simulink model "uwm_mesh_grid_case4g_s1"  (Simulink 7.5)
settings: Solver=ode45  StartTime=0.0  StopTime=8.0  RelTol=1e-4
undefined symbols (not defined in the file or in its folder): D1, Delta, dfilt, DiscIntNeverNeededParam
libraries: powerlib x90, powerlib_extras x24, dsparch4 x6
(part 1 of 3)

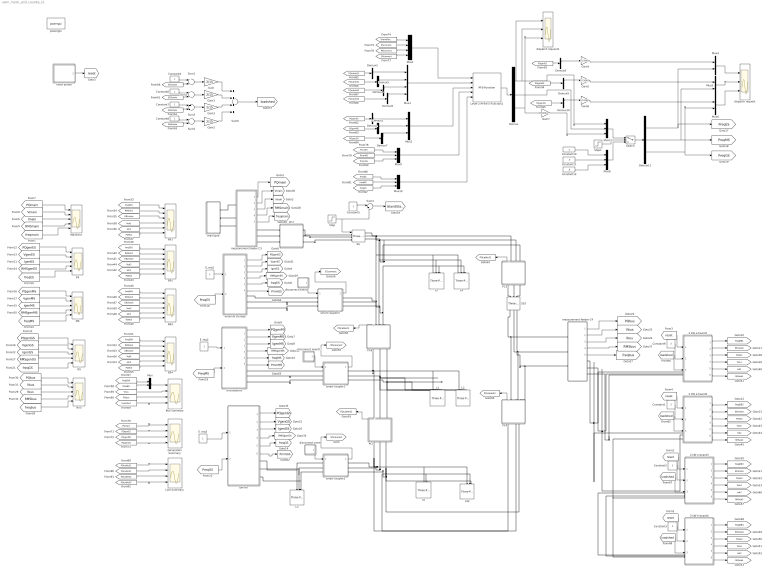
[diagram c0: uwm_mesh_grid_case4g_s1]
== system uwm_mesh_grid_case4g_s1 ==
  2 kW e-board1 : Subsystem
  2 kW e-board2 : Subsystem
  2 kW e-board3 : Subsystem
  2 kW e-board4 : Subsystem
  BUS : Scope  NumInputPorts=5
  Bus Summary : Scope  NumInputPorts=4
  Constant{1..3,9} (4 alike) : Constant  Value=2  OutDataType=fixdt(1, 16)  OutScaling=2^0
  Constant10 : Constant  Value=-.1  OutDataType=fixdt(1, 16)  OutScaling=2^0
  Constant11 : Constant  Value=.5  OutDataType=fixdt(1, 16)  OutScaling=2^0
  Constant12 : Constant  Value=.8  OutDataType=fixdt(1, 16)  OutScaling=2^0
  Constant{4..8} (5 alike) : Constant  OutDataType=fixdt(1, 16)  OutScaling=2^0
  Demux : Demux  Outputs=3
  Demux{1..10} (10 alike) : Demux  Outputs=2
  Demux11 : Demux  Outputs=3
  EB{1..4} (4 alike) : Scope  NumInputPorts=6
  ES : Scope  NumInputPorts=5
  E_req1 : Constant  OutDataType=fixdt(1, 16)  OutScaling=2^0
  E_req2 : Constant  OutDataType=fixdt(1, 16)  OutScaling=2^0
  E_req3 : Constant  OutDataType=fixdt(1, 16)  OutScaling=2^0
  GS : Scope  NumInputPorts=5
  Gain{,1..3} (4 alike) : Gain  Gain=2/15  ParameterDataType=fixdt(1, 16)  ParameterScaling=2^0  OutDataType=fixdt(1, 16)  OutScaling=2^0
  Gain4 : Gain  Gain=1/15000  ParameterDataType=fixdt(1, 16)  ParameterScaling=2^0  OutDataType=fixdt(1, 16)  OutScaling=2^0
  Gain5 : Gain  Gain=1/15000  ParameterDataType=fixdt(1, 16)  ParameterScaling=2^0  OutDataType=fixdt(1, 16)  OutScaling=2^0
  Gain6 : Gain  Gain=1/12500  ParameterDataType=fixdt(1, 16)  ParameterScaling=2^0  OutDataType=fixdt(1, 16)  OutScaling=2^0
  Gain7 : Gain  Gain=15000/12500  ParameterDataType=fixdt(1, 16)  ParameterScaling=2^0  OutDataType=fixdt(1, 16)  OutScaling=2^0
  Generation Summary : Scope  NumInputPorts=4
  L{1..4,42} (5 alike) : powerlib/Elements/Three-Phase Series RLC Load  DialogController=POWERSYS.PowerSysDialog  PhysicalDomain=powersysdomain  SubClassName=unknown  LeftPortType=p1  RightPortType=p1  LConnTagsString=A|B|C  Configuration=Y (grounded)  NominalVoltage=208  NominalFrequency=60  ActivePower=4000  InductivePower=0  CapacitivePower=0  Measurements=None
  L5 : powerlib/Elements/Three-Phase Series RLC Load  DialogController=POWERSYS.PowerSysDialog  PhysicalDomain=powersysdomain  SubClassName=unknown  LeftPortType=p1  RightPortType=p1  LConnTagsString=A|B|C  Configuration=Y (grounded)  NominalVoltage=208  NominalFrequency=60  ActivePower=2000  InductivePower=0  CapacitivePower=0  Measurements=None
  L6 : powerlib/Elements/Three-Phase Series RLC Load  DialogController=POWERSYS.PowerSysDialog  PhysicalDomain=powersysdomain  SubClassName=unknown  LeftPortType=p1  RightPortType=p1  LConnTagsString=A|B|C  Configuration=Y (grounded)  NominalVoltage=208  NominalFrequency=60  ActivePower=2000  InductivePower=0  CapacitivePower=0  Measurements=None
  Level-2 M-file S-Function1 : M-S-Function  FunctionName=dispatcher3
  Line Summary : Scope  NumInputPorts=4
  MS : Scope  NumInputPorts=5
  MainGrid : Scope  NumInputPorts=5
  Mux{,4..6} (4 alike) : Mux  Inputs=2
  Mux1 : Mux
  Mux{2,7..10} (5 alike) : Mux  Inputs=3
  Mux3 : Mux
  PC2 : Subsystem  mask{R=.002810, L=.000679, C=2894.3}
  PC3 : Subsystem  mask{R=0.027352, L=.006600, C=288.6}
  PC4 : Subsystem  mask{R=.01688, L=.004070, C=336.7}
  PC5 : Subsystem  mask{R=.002600, L=.000640, C=2020.1}
  PC6 : Subsystem  mask{R=.013700, L=.003300, C=577.2}
  SS : powerlib/Elements/Three-Phase Breaker  DialogController=POWERSYS.PowerSysDialog  SystemSampleTime=-1  InitialState=closed  SwitchA=on  SwitchB=on  SwitchC=on  SwitchTimes=[1.]  External=on  BreakerResistance=.001  SnubberResistance=1e6  SnubberCapacitance=inf  Measurements=None
  SS3 : powerlib/Elements/Three-Phase Breaker  DialogController=POWERSYS.PowerSysDialog  SystemSampleTime=-1  InitialState=closed  SwitchA=on  SwitchB=on  SwitchC=on  SwitchTimes=[50]  External=off  BreakerResistance=.00001  SnubberResistance=1e10  SnubberCapacitance=inf  Measurements=None
  Step : Step  Before=1  After=0  SampleTime=0
  Step1 : Step  Time=100  SampleTime=0
  Sum{1..3,5} (4 alike) : Sum  Inputs=+-  OutDataType=fixdt(1, 16)  OutScaling=2^0
  Sum4 : Sum  Inputs=|+-  OutDataType=fixdt(1, 16)  OutScaling=2^0
  Sum6 : Sum  Inputs=++++  OutDataType=fixdt(1, 16)  OutScaling=2^0
  Switch : Switch  Threshold=1/2  OutDataType=fixdt(1, 16)  OutScaling=2^0
  disconnect event : Subsystem  mask{tstart=50, tstop=60}
      mask prompts: tstart "disconnect time"; tstop "connect time"
  disconnect event1 : Subsystem  mask{tstart=3.0, tstop=3.5}
      mask prompts: tstart "disconnect time"; tstop "connect time"
  disconnect event2 : Subsystem  mask{tstart=50, tstop=60}
      mask prompts: tstart "disconnect time"; tstop "connect time"
  dispatch request : Scope  NumInputPorts=3
  dispatch request1 : Scope  NumInputPorts=3
  external storage : Subsystem  AncestorBlock=|
      | UWM_blocks/inverter-based
      | DG (simplified)
      | 208V - 15kVA
  genset : Subsystem
  main grid : Subsystem
  measurement feeder C3 : Subsystem
  measurement feeder C4 : Subsystem
  microsource : Subsystem  AncestorBlock=|
      | UWM_blocks/inverter-based
      | DG (simplified)
      | 208V - 15kVA
  powergui : powerlib/powergui  Priority=1  SystemSampleTime=-1  SimulationMode=Discrete  SampleTime=20e-6  frequency=60  SPID=off  DisableSnubberDevices=off  DisableRonSwitches=off  DisableVfSwitches=off  SwTol=0  Interpol=off  frequencyindice=60  echomessages=off  HookPort=off  DisplayEquations=off  FunctionMessages=off  EnableUseOfTLC=off  x0status=steady  RestoreLinks=no  ResistiveCurrentMeasurement=off  Frange=[0:2:500]  Ylog=off  Xlog=on  ShowGrid=off  save=off  variable=ZData  ZoomFFT=on  StartTime=0.0  cycles=1  DisplayStyle=1  fundamental=60  FreqAxis=off  MaxFrequency=1000  frequencyindicesteady=1  RmsSteady=2  display=off  Ts=0  methode=off
  reset pulses : Subsystem  mask{tpulse=[50 100]}
  smart coupler1 : Subsystem
  smart coupler2 : Subsystem
  smart coupler3 : Subsystem
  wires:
  [PreqMS] -> microsource/2(P_req)
  E_req2/1 -> microsource/1(E_req)
  E_req1/1 -> external storage/1(E_req)
  E_req3/1 -> genset/1(Ereq)
  [PreqGS] -> genset/2(Preq)
  reset pulses/1(Out1) -> [reset]
  2 kW e-board1/1(w) -> [freqEB1]
  2 kW e-board1/2(state) -> [EB1state]
  measurement feeder C3/3(I) -> [Imain]
  measurement feeder C3/1(PQ) -> [PQmain]
  [PreqES] -> external storage/2(P_req)
  measurement feeder C3/2(V) -> [Vmain]
  [PQmain] -> MainGrid/1
  [Vmain] -> MainGrid/2
  [Imain] -> MainGrid/3
  [RMSmain] -> MainGrid/4
  external storage/5(freq) -> [freqES]
  external storage/3(I) -> [IgenES]
  external storage/2(V) -> [VgenES]
  external storage/1(PQ) -> [PQgenES]
  microsource/1(PQ) -> [PQgenMS]
  microsource/2(V) -> [VgenMS]
  microsource/3(I) -> [IgenMS]
  microsource/5(freq) -> [freqMS]
  genset/1(PQ) -> [PQgenGS]
  genset/2(V) -> [VgenGS]
  genset/3(I) -> [IgenGS]
  genset/5(freq) -> [freqGS]
  measurement feeder C4/1(PQ) -> [PQbus]
  measurement feeder C4/2(V) -> [Vbus]
  measurement feeder C4/3(I) -> [Ibus]
  measurement feeder C4/5(freq) -> [freqbus]
  measurement feeder C3/4(RMS) -> [RMSmain]
  external storage/4(RMS) -> [RMSgenES]
  microsource/4(RMS) -> [RMSgenMS]
  genset/4(RMS) -> [RMSgenGS]
  measurement feeder C3/5(freq) -> [freqmain]
  [freqmain] -> MainGrid/5
  [PQgenES] -> ES/1
  [VgenES] -> ES/2
  [IgenES] -> ES/3
  [RMSgenES] -> ES/4
  [freqES] -> ES/5
  [PQgenMS] -> MS/1
  [VgenMS] -> MS/2
  [IgenMS] -> MS/3
  [RMSgenMS] -> MS/4
  [freqMS] -> MS/5
  [PQgenGS] -> GS/1
  [VgenGS] -> GS/2
  [IgenGS] -> GS/3
  [RMSgenGS] -> GS/4
  [freqGS] -> GS/5
  measurement feeder C4/4(RMS) -> [RMSbus]
  [PQbus] -> BUS/1
  [Vbus] -> BUS/2
  [Ibus] -> BUS/3
  [RMSbus] -> BUS/4
  [freqbus] -> BUS/5
  [freqEB1] -> EB1/1
  [RMSeb1] -> EB1/2
  [EB1state] -> EB1/3
  2 kW e-board1/3(PQ) -> [PQeb1]
  2 kW e-board1/4(V) -> [Veb1]
  2 kW e-board1/5(I) -> [Ieb1]
  2 kW e-board1/6(RMS) -> [RMSeb1]
  [PQeb1] -> EB1/6
  [Ieb1] -> EB1/5
  [Veb1] -> EB1/4
  [reset] -> 2 kW e-board2/1(reset)
  2 kW e-board2/1(w) -> [freqEB2]
  2 kW e-board2/2(state) -> [EB2state]
  Constant1/1 -> 2 kW e-board2/2(priority)
  2 kW e-board2/3(PQ) -> [PQeb2]
  2 kW e-board2/4(V) -> [Veb2]
  2 kW e-board2/5(I) -> [Ieb2]
  2 kW e-board2/6(RMS) -> [RMSeb2]
  2 kW e-board3/1(w) -> [freqEB3]
  2 kW e-board3/2(state) -> [EB3state]
  2 kW e-board3/3(PQ) -> [PQeb3]
  2 kW e-board3/4(V) -> [Veb3]
  2 kW e-board3/5(I) -> [Ieb3]
  2 kW e-board3/6(RMS) -> [RMSeb3]
  2 kW e-board4/1(w) -> [freqEB4]
  2 kW e-board4/2(state) -> [EB4state]
  2 kW e-board4/3(PQ) -> [PQeb4]
  2 kW e-board4/4(V) -> [Veb4]
  2 kW e-board4/5(I) -> [Ieb4]
  2 kW e-board4/6(RMS) -> [RMSeb4]
  [freqEB2] -> EB2/1
  [RMSeb2] -> EB2/2
  [EB2state] -> EB2/3
  [PQeb2] -> EB2/6
  [Ieb2] -> EB2/5
  [Veb2] -> EB2/4
  [freqEB3] -> EB3/1
  [RMSeb3] -> EB3/2
  [EB3state] -> EB3/3
  [PQeb3] -> EB3/6
  [Ieb3] -> EB3/5
  [Veb3] -> EB3/4
  [freqEB4] -> EB4/1
  [RMSeb4] -> EB4/2
  [EB4state] -> EB4/3
  [PQeb4] -> EB4/6
  [Ieb4] -> EB4/5
  [Veb4] -> EB4/4
  Step/1 -> SS/1, Sum4/2
  [freqEB4] -> Mux/1
  [freqES] -> Mux/2
  [PQbus] -> Bus Summary/3
  Mux/1 -> Bus Summary/1
  [Vbus] -> Bus Summary/2
  disconnect event/1(Out1) -> smart coupler2/1(event)
  smart coupler2/1(connected) -> [GSconnect]
  Constant5/1 -> Sum4/1
  Sum4/1 -> [IslandState]
  disconnect event1/1(Out1) -> smart coupler1/1(event)
  smart coupler1/1(connected) -> [MSconnect]
  disconnect event2/1(Out1) -> smart coupler3/1(event)
  smart coupler3/1(connected) -> [ESconnect]
  Constant4/1 -> Sum1/1
  [EB1state] -> Sum1/2
  Constant6/1 -> Sum2/1
  [EB2state] -> Sum2/2
  Constant7/1 -> Sum3/1
  [EB3state] -> Sum3/2
  Constant8/1 -> Sum5/1
  [EB4state] -> Sum5/2
  Sum1/1 -> Gain/1
  Sum2/1 -> Gain1/1
  Sum3/1 -> Gain3/1
  Sum5/1 -> Gain2/1
  Gain1/1 -> Sum6/2
  Gain3/1 -> Sum6/3
  Gain/1 -> Sum6/1
  Gain2/1 -> Sum6/4
  Sum6/1 -> [loadshed]
  [loadshed] -> 2 kW e-board2/3(shed_load)
  [reset] -> 2 kW e-board1/1(reset)
  Constant9/1 -> 2 kW e-board1/2(priority)
  [loadshed] -> 2 kW e-board1/3(shed_load)
  [reset] -> 2 kW e-board3/1(reset)
  Constant2/1 -> 2 kW e-board3/2(priority)
  [loadshed] -> 2 kW e-board3/3(shed_load)
  [reset] -> 2 kW e-board4/1(reset)
  Constant3/1 -> 2 kW e-board4/2(priority)
  [loadshed] -> 2 kW e-board4/3(shed_load)
  [loadshed] -> Bus Summary/4
  [PQgenES] -> Generation Summary/2
  [PQgenMS] -> Generation Summary/3
  [PQmain] -> Generation Summary/1
  [PQgenGS] -> Generation Summary/4
  [GSconnect] -> Mux1/4
  [MSconnect] -> Mux1/3
  [ESconnect] -> Mux1/2
  [IslandState] -> Mux1/1
  PC6/1(PQ) -> [PQcable21]
  PC5/1(PQ) -> [PQcable42]
  PC4/1(PQ) -> [PQcable43]
  PC3/1(PQ) -> [PQcable31]
  [PQcable31] -> Demux4/1
  [PQcable42] -> Demux5/1
  [PQcable21] -> Demux3/1
  [PQcable43] -> Demux6/1
  Demux3/1 -> Mux3/1
  Demux4/1 -> Mux3/2
  Demux5/1 -> Mux3/3
  Demux6/1 -> Mux3/4
  Mux1/1 -> Level-2 M-file S-Function1/1
  Mux3/1 -> Level-2 M-file S-Function1/2
  Level-2 M-file S-Function1/1 -> Demux/1
  [PQgenMS] -> Demux2/1
  [PQgenGS] -> Demux7/1
  [PQgenES] -> Demux1/1
  Mux2/1 -> Level-2 M-file S-Function1/3
  [PQcable21] -> Line Summary/1
  [PQcable31] -> Line Summary/2
  [PQcable42] -> Line Summary/3
  [PQcable43] -> Line Summary/4
  [PQgenMS] -> Demux9/1
  [PQgenGS] -> Demux10/1
  [PQgenES] -> Demux8/1
  Demux/1 -> dispatch request1/1, Mux7/1, dispatch request1/2
  Demux/2 -> Mux7/2
  Demux8/1 -> Gain4/1
  Gain4/1 -> Mux4/1
  Demux9/1 -> Gain5/1
  Gain5/1 -> Mux5/1
  Demux10/1 -> Gain6/1
  Gain6/1 -> Mux6/1
  Constant10/1 -> Mux8/1
  Constant11/1 -> Mux8/2
  Constant12/1 -> Mux8/3
  Mux8/1 -> Switch/3
  Mux7/1 -> Switch/1
  Switch/1 -> Demux11/1
  Step1/1 -> Switch/2
  genset/6(Pmm) -> [PmmGS]
  microsource/6(Pmm) -> [PmmMS]
  external storage/6(Pmm) -> [PmmES]
  [PmmES] -> Mux9/1
  [PmmMS] -> Mux9/2
  [PmmGS] -> Mux9/3
  Mux9/1 -> Level-2 M-file S-Function1/4
  Demux11/1 -> [PreqES], Mux4/2
  Demux11/2 -> [PreqMS], Mux5/2
  Demux11/3 -> [PreqGS], Mux6/2
  Mux4/1 -> dispatch request/1
  Mux5/1 -> dispatch request/2
  Mux6/1 -> dispatch request/3
  Demux/3 -> Gain7/1, dispatch request1/3
  Gain7/1 -> Mux7/3
  Demux1/1 -> Mux2/1
  Demux2/1 -> Mux2/2
  Demux7/1 -> Mux2/3
  [freqES] -> Mux10/1
  [freqMS] -> Mux10/2
  [freqGS] -> Mux10/3
  Mux10/1 -> Level-2 M-file S-Function1/5
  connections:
  measurement feeder C4/LConn1 -- PC4/RConn1 -- SS3/RConn1
  measurement feeder C4/LConn2 -- PC4/RConn2 -- SS3/RConn2
  measurement feeder C4/LConn3 -- PC4/RConn3 -- SS3/RConn3
  L42/LConn1 -- PC5/LConn1 -- PC4/LConn1 -- smart coupler2/RConn1 -- L6/LConn1
  L42/LConn3 -- PC4/LConn3 -- PC5/LConn3 -- smart coupler2/RConn3 -- L6/LConn3
  PC5/RConn1 -- L1/LConn1 -- L2/LConn1 -- PC6/LConn1 -- smart coupler1/RConn1
  L2/LConn2 -- L1/LConn2 -- PC5/RConn2 -- PC6/LConn2 -- smart coupler1/RConn2
  L2/LConn3 -- L1/LConn3 -- PC5/RConn3 -- PC6/LConn3 -- smart coupler1/RConn3
  main grid/RConn2 -- measurement feeder C3/LConn2
  main grid/RConn1 -- measurement feeder C3/LConn1
  measurement feeder C3/LConn3 -- main grid/RConn3
  measurement feeder C3/RConn1 -- PC2/LConn1
  measurement feeder C3/RConn2 -- PC2/LConn2
  measurement feeder C3/RConn3 -- PC2/LConn3
  PC2/RConn2 -- SS/LConn2
  PC2/RConn1 -- SS/LConn1
  SS/LConn3 -- PC2/RConn3
  SS3/LConn2 -- PC3/LConn2
  SS3/LConn3 -- PC3/LConn3
  SS3/LConn1 -- PC3/LConn1
  L5/LConn1 -- genset/RConn1 -- smart coupler2/LConn1
  L5/LConn2 -- genset/RConn2 -- smart coupler2/LConn2
  L5/LConn3 -- genset/RConn3 -- smart coupler2/LConn3
  2 kW e-board4/LConn2 -- measurement feeder C4/RConn2 -- 2 kW e-board1/LConn2 -- 2 kW e-board2/LConn2 -- 2 kW e-board3/LConn2
  2 kW e-board3/LConn3 -- measurement feeder C4/RConn3 -- 2 kW e-board1/LConn3 -- 2 kW e-board2/LConn3 -- 2 kW e-board4/LConn3
  2 kW e-board4/LConn1 -- measurement feeder C4/RConn1 -- 2 kW e-board1/LConn1 -- 2 kW e-board2/LConn1 -- 2 kW e-board3/LConn1
  PC6/RConn1 -- L3/LConn1 -- L4/LConn1 -- SS/RConn1 -- PC3/RConn1 -- smart coupler3/RConn1
  PC6/RConn2 -- L3/LConn2 -- L4/LConn2 -- SS/RConn2 -- PC3/RConn2 -- smart coupler3/RConn2
  PC6/RConn3 -- L3/LConn3 -- L4/LConn3 -- SS/RConn3 -- PC3/RConn3 -- smart coupler3/RConn3
  L42/LConn2 -- PC5/LConn2 -- smart coupler2/RConn2 -- PC4/LConn2 -- L6/LConn2
  microsource/RConn1 -- smart coupler1/LConn1
  smart coupler1/LConn2 -- microsource/RConn2
  smart coupler1/LConn3 -- microsource/RConn3
  smart coupler3/LConn1 -- external storage/RConn1
  smart coupler3/LConn2 -- external storage/RConn2
  smart coupler3/LConn3 -- external storage/RConn3

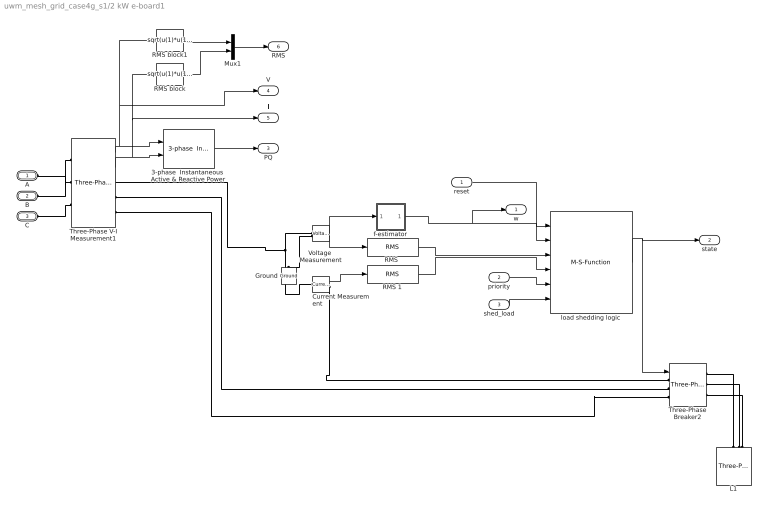
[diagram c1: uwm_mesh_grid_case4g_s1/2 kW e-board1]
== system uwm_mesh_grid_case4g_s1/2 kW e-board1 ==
  reset : Inport
  priority : Inport  Port=2
  shed_load : Inport  Port=3
  3-phase  Instantaneous  Active & Reactive Power : powerlib_extras/Measurements/3-phase  Instantaneous  Active & Reactive Power  DialogController=POWERSYS.PowerSysDialog  SystemSampleTime=-1
  Current Measurement : powerlib/Measurements/Current Measurement  DialogController=POWERSYS.PowerSysDialog  SystemSampleTime=-1  PhasorSimulation=off  OutputType=Complex  PSBequivalent=0
  Ground : powerlib/Elements/Ground  DialogController=POWERSYS.PowerSysDialog  PhysicalDomain=powersysdomain  SubClassName=unknown  LeftPortType=p1  RightPortType=p1  LConnTagsString=a
  L1 : powerlib/Elements/Three-Phase Series RLC Load  DialogController=POWERSYS.PowerSysDialog  PhysicalDomain=powersysdomain  SubClassName=unknown  LeftPortType=p1  RightPortType=p1  LConnTagsString=A|B|C  Configuration=Y (grounded)  NominalVoltage=208  NominalFrequency=60  ActivePower=2000  InductivePower=0  CapacitivePower=0  Measurements=None
  Mux1 : Mux  Inputs=2
  "RMS " : powerlib_extras/Measurements/RMS  DialogController=POWERSYS.PowerSysDialog  SystemSampleTime=-1  f1=60
  RMS 1 : powerlib_extras/Measurements/RMS  DialogController=POWERSYS.PowerSysDialog  SystemSampleTime=-1  f1=60
  RMS block : Fcn  Expr=sqrt(u(1)*u(1)+u(2)*u(2)+u(3)*u(3))/sqrt(3)
  RMS block1 : Fcn  Expr=sqrt(u(1)*u(1)+u(2)*u(2)+u(3)*u(3))/sqrt(3)
  Three-Phase V-I Measurement1 : powerlib/Measurements/Three-Phase V-I Measurement  DialogController=POWERSYS.PowerSysDialog  SystemSampleTime=-1  VoltageMeasurement=phase-to-ground  SetLabelV=off  LabelV=Vabc  Vpu=off  VpuLL=off  CurrentMeasurement=yes  SetLabelI=off  LabelI=Iabc  Ipu=off  Pbase=100e6  Vbase=500e3  OutputType=Complex  PhasorSimulation=off  PSBequivalent=0
  Three-Phase Breaker2 : powerlib/Elements/Three-Phase Breaker  DialogController=POWERSYS.PowerSysDialog  SystemSampleTime=-1  InitialState=closed  SwitchA=on  SwitchB=on  SwitchC=on  SwitchTimes=[50]  External=on  BreakerResistance=0.001  SnubberResistance=1e6  SnubberCapacitance=inf  Measurements=None
  Voltage  Measurement : powerlib/Measurements/Voltage Measurement  DialogController=POWERSYS.PowerSysDialog  SystemSampleTime=-1  PhasorSimulation=off  OutputType=Complex  PSBequivalent=0
  f-estimator : Subsystem  mask{dt=0.010}
      mask prompts: dt "sample time"
  load shedding logic : M-S-Function  FunctionName=load_shedding_logic3
  A : PMIOPort  Port=1  Side=Left
  B : PMIOPort  Port=2  Side=Left
  C : PMIOPort  Port=3  Side=Left
  w : Outport  OutDataType=fixdt(1, 16)  OutScaling=2^0
  state : Outport  Port=2  OutDataType=fixdt(1, 16)  OutScaling=2^0
  PQ : Outport  Port=3  OutDataType=fixdt(1, 16)  OutScaling=2^0
  V : Outport  Port=4  OutDataType=fixdt(1, 16)  OutScaling=2^0
  I : Outport  Port=5  OutDataType=fixdt(1, 16)  OutScaling=2^0
  RMS : Outport  Port=6  OutDataType=fixdt(1, 16)  OutScaling=2^0
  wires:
  reset/1 -> load shedding logic/1
  Current Measurement/1 -> RMS 1/1
  Voltage  Measurement/1 -> "RMS "/1, f-estimator/1(v)
  f-estimator/1(w) -> load shedding logic/2, w/1
  "RMS "/1 -> load shedding logic/3
  RMS 1/1 -> load shedding logic/4
  load shedding logic/1 -> Three-Phase Breaker2/1, state/1
  priority/1 -> load shedding logic/5
  Three-Phase V-I Measurement1/1 -> 3-phase  Instantaneous  Active & Reactive Power/1, RMS block1/1, V/1
  Three-Phase V-I Measurement1/2 -> 3-phase  Instantaneous  Active & Reactive Power/2, RMS block/1, I/1
  3-phase  Instantaneous  Active & Reactive Power/1 -> PQ/1
  RMS block1/1 -> Mux1/1
  RMS block/1 -> Mux1/2
  Mux1/1 -> RMS/1
  shed_load/1 -> load shedding logic/6
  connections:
  Voltage  Measurement/LConn1 -- Current Measurement/LConn1 -- Three-Phase V-I Measurement1/RConn1
  Voltage  Measurement/LConn2 -- Ground/LConn1
  Current Measurement/RConn1 -- Three-Phase Breaker2/LConn1
  L1/LConn1 -- Three-Phase Breaker2/RConn1
  L1/LConn2 -- Three-Phase Breaker2/RConn2
  L1/LConn3 -- Three-Phase Breaker2/RConn3
  Three-Phase V-I Measurement1/LConn1 -- A/RConn1
  Three-Phase V-I Measurement1/LConn2 -- B/RConn1
  Three-Phase V-I Measurement1/LConn3 -- C/RConn1
  Three-Phase V-I Measurement1/RConn2 -- Three-Phase Breaker2/LConn2
  Three-Phase V-I Measurement1/RConn3 -- Three-Phase Breaker2/LConn3

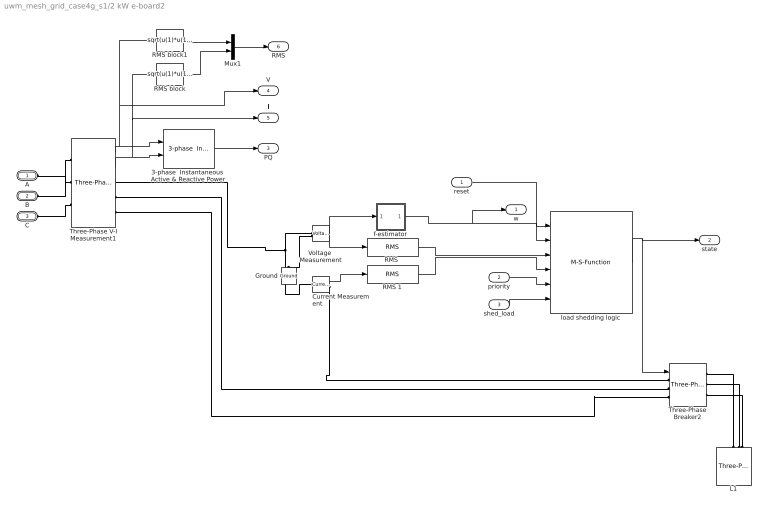
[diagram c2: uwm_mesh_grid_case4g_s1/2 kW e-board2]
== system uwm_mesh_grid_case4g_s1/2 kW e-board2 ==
  reset : Inport
  priority : Inport  Port=2
  shed_load : Inport  Port=3
  3-phase  Instantaneous  Active & Reactive Power : powerlib_extras/Measurements/3-phase  Instantaneous  Active & Reactive Power  DialogController=POWERSYS.PowerSysDialog  SystemSampleTime=-1
  Current Measurement : powerlib/Measurements/Current Measurement  DialogController=POWERSYS.PowerSysDialog  SystemSampleTime=-1  PhasorSimulation=off  OutputType=Complex  PSBequivalent=0
  Ground : powerlib/Elements/Ground  DialogController=POWERSYS.PowerSysDialog  PhysicalDomain=powersysdomain  SubClassName=unknown  LeftPortType=p1  RightPortType=p1  LConnTagsString=a
  L1 : powerlib/Elements/Three-Phase Series RLC Load  DialogController=POWERSYS.PowerSysDialog  PhysicalDomain=powersysdomain  SubClassName=unknown  LeftPortType=p1  RightPortType=p1  LConnTagsString=A|B|C  Configuration=Y (grounded)  NominalVoltage=208  NominalFrequency=60  ActivePower=2000  InductivePower=0  CapacitivePower=0  Measurements=None
  Mux1 : Mux  Inputs=2
  "RMS " : powerlib_extras/Measurements/RMS  DialogController=POWERSYS.PowerSysDialog  SystemSampleTime=-1  f1=60
  RMS 1 : powerlib_extras/Measurements/RMS  DialogController=POWERSYS.PowerSysDialog  SystemSampleTime=-1  f1=60
  RMS block : Fcn  Expr=sqrt(u(1)*u(1)+u(2)*u(2)+u(3)*u(3))/sqrt(3)
  RMS block1 : Fcn  Expr=sqrt(u(1)*u(1)+u(2)*u(2)+u(3)*u(3))/sqrt(3)
  Three-Phase V-I Measurement1 : powerlib/Measurements/Three-Phase V-I Measurement  DialogController=POWERSYS.PowerSysDialog  SystemSampleTime=-1  VoltageMeasurement=phase-to-ground  SetLabelV=off  LabelV=Vabc  Vpu=off  VpuLL=off  CurrentMeasurement=yes  SetLabelI=off  LabelI=Iabc  Ipu=off  Pbase=100e6  Vbase=500e3  OutputType=Complex  PhasorSimulation=off  PSBequivalent=0
  Three-Phase Breaker2 : powerlib/Elements/Three-Phase Breaker  DialogController=POWERSYS.PowerSysDialog  SystemSampleTime=-1  InitialState=closed  SwitchA=on  SwitchB=on  SwitchC=on  SwitchTimes=[50]  External=on  BreakerResistance=0.001  SnubberResistance=1e6  SnubberCapacitance=inf  Measurements=None
  Voltage  Measurement : powerlib/Measurements/Voltage Measurement  DialogController=POWERSYS.PowerSysDialog  SystemSampleTime=-1  PhasorSimulation=off  OutputType=Complex  PSBequivalent=0
  f-estimator : Subsystem  mask{dt=0.010}
      mask prompts: dt "sample time"
  load shedding logic : M-S-Function  FunctionName=load_shedding_logic3
  A : PMIOPort  Port=1  Side=Left
  B : PMIOPort  Port=2  Side=Left
  C : PMIOPort  Port=3  Side=Left
  w : Outport  OutDataType=fixdt(1, 16)  OutScaling=2^0
  state : Outport  Port=2  OutDataType=fixdt(1, 16)  OutScaling=2^0
  PQ : Outport  Port=3  OutDataType=fixdt(1, 16)  OutScaling=2^0
  V : Outport  Port=4  OutDataType=fixdt(1, 16)  OutScaling=2^0
  I : Outport  Port=5  OutDataType=fixdt(1, 16)  OutScaling=2^0
  RMS : Outport  Port=6  OutDataType=fixdt(1, 16)  OutScaling=2^0
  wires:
  reset/1 -> load shedding logic/1
  Current Measurement/1 -> RMS 1/1
  Voltage  Measurement/1 -> "RMS "/1, f-estimator/1(v)
  f-estimator/1(w) -> load shedding logic/2, w/1
  "RMS "/1 -> load shedding logic/3
  RMS 1/1 -> load shedding logic/4
  load shedding logic/1 -> Three-Phase Breaker2/1, state/1
  priority/1 -> load shedding logic/5
  Three-Phase V-I Measurement1/1 -> 3-phase  Instantaneous  Active & Reactive Power/1, RMS block1/1, V/1
  Three-Phase V-I Measurement1/2 -> 3-phase  Instantaneous  Active & Reactive Power/2, RMS block/1, I/1
  3-phase  Instantaneous  Active & Reactive Power/1 -> PQ/1
  RMS block1/1 -> Mux1/1
  RMS block/1 -> Mux1/2
  Mux1/1 -> RMS/1
  shed_load/1 -> load shedding logic/6
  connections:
  Voltage  Measurement/LConn1 -- Current Measurement/LConn1 -- Three-Phase V-I Measurement1/RConn1
  Voltage  Measurement/LConn2 -- Ground/LConn1
  Current Measurement/RConn1 -- Three-Phase Breaker2/LConn1
  L1/LConn1 -- Three-Phase Breaker2/RConn1
  L1/LConn2 -- Three-Phase Breaker2/RConn2
  L1/LConn3 -- Three-Phase Breaker2/RConn3
  Three-Phase V-I Measurement1/LConn1 -- A/RConn1
  Three-Phase V-I Measurement1/LConn2 -- B/RConn1
  Three-Phase V-I Measurement1/LConn3 -- C/RConn1
  Three-Phase V-I Measurement1/RConn2 -- Three-Phase Breaker2/LConn2
  Three-Phase V-I Measurement1/RConn3 -- Three-Phase Breaker2/LConn3

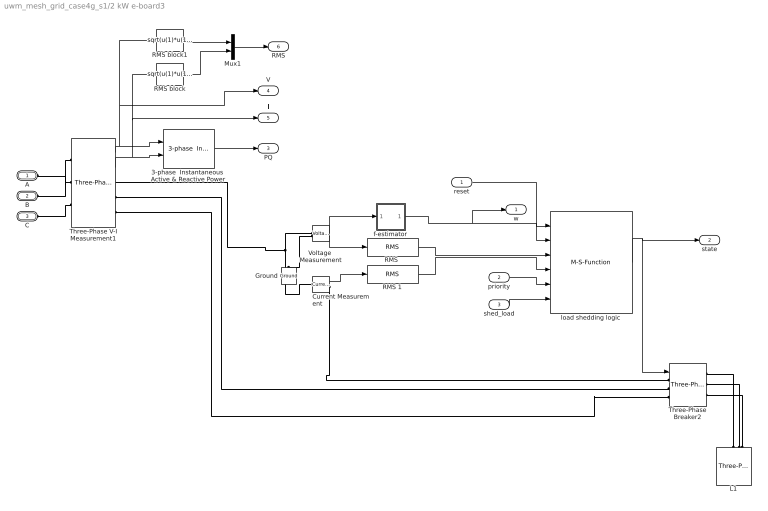
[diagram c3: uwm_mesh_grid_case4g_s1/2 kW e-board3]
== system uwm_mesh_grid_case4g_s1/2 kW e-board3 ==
  reset : Inport
  priority : Inport  Port=2
  shed_load : Inport  Port=3
  3-phase  Instantaneous  Active & Reactive Power : powerlib_extras/Measurements/3-phase  Instantaneous  Active & Reactive Power  DialogController=POWERSYS.PowerSysDialog  SystemSampleTime=-1
  Current Measurement : powerlib/Measurements/Current Measurement  DialogController=POWERSYS.PowerSysDialog  SystemSampleTime=-1  PhasorSimulation=off  OutputType=Complex  PSBequivalent=0
  Ground : powerlib/Elements/Ground  DialogController=POWERSYS.PowerSysDialog  PhysicalDomain=powersysdomain  SubClassName=unknown  LeftPortType=p1  RightPortType=p1  LConnTagsString=a
  L1 : powerlib/Elements/Three-Phase Series RLC Load  DialogController=POWERSYS.PowerSysDialog  PhysicalDomain=powersysdomain  SubClassName=unknown  LeftPortType=p1  RightPortType=p1  LConnTagsString=A|B|C  Configuration=Y (grounded)  NominalVoltage=208  NominalFrequency=60  ActivePower=2000  InductivePower=0  CapacitivePower=0  Measurements=None
  Mux1 : Mux  Inputs=2
  "RMS " : powerlib_extras/Measurements/RMS  DialogController=POWERSYS.PowerSysDialog  SystemSampleTime=-1  f1=60
  RMS 1 : powerlib_extras/Measurements/RMS  DialogController=POWERSYS.PowerSysDialog  SystemSampleTime=-1  f1=60
  RMS block : Fcn  Expr=sqrt(u(1)*u(1)+u(2)*u(2)+u(3)*u(3))/sqrt(3)
  RMS block1 : Fcn  Expr=sqrt(u(1)*u(1)+u(2)*u(2)+u(3)*u(3))/sqrt(3)
  Three-Phase V-I Measurement1 : powerlib/Measurements/Three-Phase V-I Measurement  DialogController=POWERSYS.PowerSysDialog  SystemSampleTime=-1  VoltageMeasurement=phase-to-ground  SetLabelV=off  LabelV=Vabc  Vpu=off  VpuLL=off  CurrentMeasurement=yes  SetLabelI=off  LabelI=Iabc  Ipu=off  Pbase=100e6  Vbase=500e3  OutputType=Complex  PhasorSimulation=off  PSBequivalent=0
  Three-Phase Breaker2 : powerlib/Elements/Three-Phase Breaker  DialogController=POWERSYS.PowerSysDialog  SystemSampleTime=-1  InitialState=closed  SwitchA=on  SwitchB=on  SwitchC=on  SwitchTimes=[50]  External=on  BreakerResistance=0.001  SnubberResistance=1e6  SnubberCapacitance=inf  Measurements=None
  Voltage  Measurement : powerlib/Measurements/Voltage Measurement  DialogController=POWERSYS.PowerSysDialog  SystemSampleTime=-1  PhasorSimulation=off  OutputType=Complex  PSBequivalent=0
  f-estimator : Subsystem  mask{dt=0.010}
      mask prompts: dt "sample time"
  load shedding logic : M-S-Function  FunctionName=load_shedding_logic3
  A : PMIOPort  Port=1  Side=Left
  B : PMIOPort  Port=2  Side=Left
  C : PMIOPort  Port=3  Side=Left
  w : Outport  OutDataType=fixdt(1, 16)  OutScaling=2^0
  state : Outport  Port=2  OutDataType=fixdt(1, 16)  OutScaling=2^0
  PQ : Outport  Port=3  OutDataType=fixdt(1, 16)  OutScaling=2^0
  V : Outport  Port=4  OutDataType=fixdt(1, 16)  OutScaling=2^0
  I : Outport  Port=5  OutDataType=fixdt(1, 16)  OutScaling=2^0
  RMS : Outport  Port=6  OutDataType=fixdt(1, 16)  OutScaling=2^0
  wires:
  reset/1 -> load shedding logic/1
  Current Measurement/1 -> RMS 1/1
  Voltage  Measurement/1 -> "RMS "/1, f-estimator/1(v)
  f-estimator/1(w) -> load shedding logic/2, w/1
  "RMS "/1 -> load shedding logic/3
  RMS 1/1 -> load shedding logic/4
  load shedding logic/1 -> Three-Phase Breaker2/1, state/1
  priority/1 -> load shedding logic/5
  Three-Phase V-I Measurement1/1 -> 3-phase  Instantaneous  Active & Reactive Power/1, RMS block1/1, V/1
  Three-Phase V-I Measurement1/2 -> 3-phase  Instantaneous  Active & Reactive Power/2, RMS block/1, I/1
  3-phase  Instantaneous  Active & Reactive Power/1 -> PQ/1
  RMS block1/1 -> Mux1/1
  RMS block/1 -> Mux1/2
  Mux1/1 -> RMS/1
  shed_load/1 -> load shedding logic/6
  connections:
  Voltage  Measurement/LConn1 -- Current Measurement/LConn1 -- Three-Phase V-I Measurement1/RConn1
  Voltage  Measurement/LConn2 -- Ground/LConn1
  Current Measurement/RConn1 -- Three-Phase Breaker2/LConn1
  L1/LConn1 -- Three-Phase Breaker2/RConn1
  L1/LConn2 -- Three-Phase Breaker2/RConn2
  L1/LConn3 -- Three-Phase Breaker2/RConn3
  Three-Phase V-I Measurement1/LConn1 -- A/RConn1
  Three-Phase V-I Measurement1/LConn2 -- B/RConn1
  Three-Phase V-I Measurement1/LConn3 -- C/RConn1
  Three-Phase V-I Measurement1/RConn2 -- Three-Phase Breaker2/LConn2
  Three-Phase V-I Measurement1/RConn3 -- Three-Phase Breaker2/LConn3

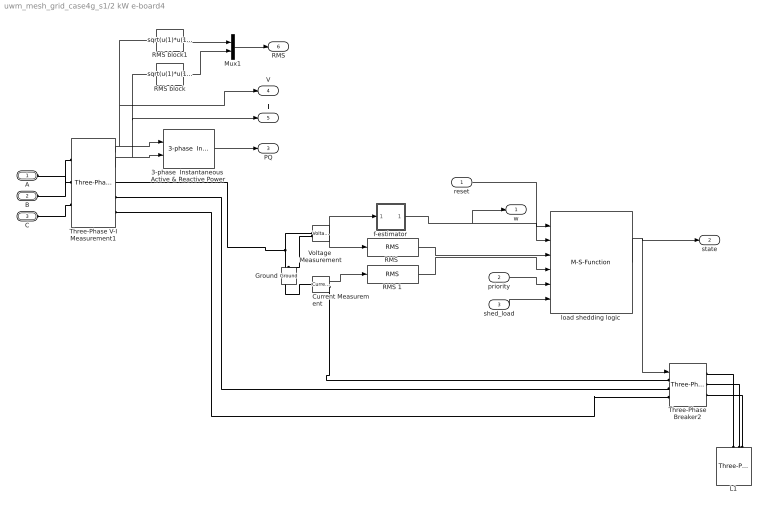
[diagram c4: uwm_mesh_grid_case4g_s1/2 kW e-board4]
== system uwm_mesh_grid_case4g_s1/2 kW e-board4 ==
  reset : Inport
  priority : Inport  Port=2
  shed_load : Inport  Port=3
  3-phase  Instantaneous  Active & Reactive Power : powerlib_extras/Measurements/3-phase  Instantaneous  Active & Reactive Power  DialogController=POWERSYS.PowerSysDialog  SystemSampleTime=-1
  Current Measurement : powerlib/Measurements/Current Measurement  DialogController=POWERSYS.PowerSysDialog  SystemSampleTime=-1  PhasorSimulation=off  OutputType=Complex  PSBequivalent=0
  Ground : powerlib/Elements/Ground  DialogController=POWERSYS.PowerSysDialog  PhysicalDomain=powersysdomain  SubClassName=unknown  LeftPortType=p1  RightPortType=p1  LConnTagsString=a
  L1 : powerlib/Elements/Three-Phase Series RLC Load  DialogController=POWERSYS.PowerSysDialog  PhysicalDomain=powersysdomain  SubClassName=unknown  LeftPortType=p1  RightPortType=p1  LConnTagsString=A|B|C  Configuration=Y (grounded)  NominalVoltage=208  NominalFrequency=60  ActivePower=2000  InductivePower=0  CapacitivePower=0  Measurements=None
  Mux1 : Mux  Inputs=2
  "RMS " : powerlib_extras/Measurements/RMS  DialogController=POWERSYS.PowerSysDialog  SystemSampleTime=-1  f1=60
  RMS 1 : powerlib_extras/Measurements/RMS  DialogController=POWERSYS.PowerSysDialog  SystemSampleTime=-1  f1=60
  RMS block : Fcn  Expr=sqrt(u(1)*u(1)+u(2)*u(2)+u(3)*u(3))/sqrt(3)
  RMS block1 : Fcn  Expr=sqrt(u(1)*u(1)+u(2)*u(2)+u(3)*u(3))/sqrt(3)
  Three-Phase V-I Measurement1 : powerlib/Measurements/Three-Phase V-I Measurement  DialogController=POWERSYS.PowerSysDialog  SystemSampleTime=-1  VoltageMeasurement=phase-to-ground  SetLabelV=off  LabelV=Vabc  Vpu=off  VpuLL=off  CurrentMeasurement=yes  SetLabelI=off  LabelI=Iabc  Ipu=off  Pbase=100e6  Vbase=500e3  OutputType=Complex  PhasorSimulation=off  PSBequivalent=0
  Three-Phase Breaker2 : powerlib/Elements/Three-Phase Breaker  DialogController=POWERSYS.PowerSysDialog  SystemSampleTime=-1  InitialState=closed  SwitchA=on  SwitchB=on  SwitchC=on  SwitchTimes=[50]  External=on  BreakerResistance=0.001  SnubberResistance=1e6  SnubberCapacitance=inf  Measurements=None
  Voltage  Measurement : powerlib/Measurements/Voltage Measurement  DialogController=POWERSYS.PowerSysDialog  SystemSampleTime=-1  PhasorSimulation=off  OutputType=Complex  PSBequivalent=0
  f-estimator : Subsystem  mask{dt=0.010}
      mask prompts: dt "sample time"
  load shedding logic : M-S-Function  FunctionName=load_shedding_logic3
  A : PMIOPort  Port=1  Side=Left
  B : PMIOPort  Port=2  Side=Left
  C : PMIOPort  Port=3  Side=Left
  w : Outport  OutDataType=fixdt(1, 16)  OutScaling=2^0
  state : Outport  Port=2  OutDataType=fixdt(1, 16)  OutScaling=2^0
  PQ : Outport  Port=3  OutDataType=fixdt(1, 16)  OutScaling=2^0
  V : Outport  Port=4  OutDataType=fixdt(1, 16)  OutScaling=2^0
  I : Outport  Port=5  OutDataType=fixdt(1, 16)  OutScaling=2^0
  RMS : Outport  Port=6  OutDataType=fixdt(1, 16)  OutScaling=2^0
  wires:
  reset/1 -> load shedding logic/1
  Current Measurement/1 -> RMS 1/1
  Voltage  Measurement/1 -> "RMS "/1, f-estimator/1(v)
  f-estimator/1(w) -> load shedding logic/2, w/1
  "RMS "/1 -> load shedding logic/3
  RMS 1/1 -> load shedding logic/4
  load shedding logic/1 -> Three-Phase Breaker2/1, state/1
  priority/1 -> load shedding logic/5
  Three-Phase V-I Measurement1/1 -> 3-phase  Instantaneous  Active & Reactive Power/1, RMS block1/1, V/1
  Three-Phase V-I Measurement1/2 -> 3-phase  Instantaneous  Active & Reactive Power/2, RMS block/1, I/1
  3-phase  Instantaneous  Active & Reactive Power/1 -> PQ/1
  RMS block1/1 -> Mux1/1
  RMS block/1 -> Mux1/2
  Mux1/1 -> RMS/1
  shed_load/1 -> load shedding logic/6
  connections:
  Voltage  Measurement/LConn1 -- Current Measurement/LConn1 -- Three-Phase V-I Measurement1/RConn1
  Voltage  Measurement/LConn2 -- Ground/LConn1
  Current Measurement/RConn1 -- Three-Phase Breaker2/LConn1
  L1/LConn1 -- Three-Phase Breaker2/RConn1
  L1/LConn2 -- Three-Phase Breaker2/RConn2
  L1/LConn3 -- Three-Phase Breaker2/RConn3
  Three-Phase V-I Measurement1/LConn1 -- A/RConn1
  Three-Phase V-I Measurement1/LConn2 -- B/RConn1
  Three-Phase V-I Measurement1/LConn3 -- C/RConn1
  Three-Phase V-I Measurement1/RConn2 -- Three-Phase Breaker2/LConn2
  Three-Phase V-I Measurement1/RConn3 -- Three-Phase Breaker2/LConn3

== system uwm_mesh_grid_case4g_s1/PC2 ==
  Ground : powerlib/Elements/Ground  DialogController=POWERSYS.PowerSysDialog  PhysicalDomain=powersysdomain  SubClassName=unknown  LeftPortType=p1  RightPortType=p1  LConnTagsString=a
  Three-Phase Parallel RLC Branch : powerlib/Elements/Three-Phase Parallel RLC Branch  DialogController=POWERSYS.PowerSysDialog  PhysicalDomain=powersysdomain  SubClassName=unknown  LeftPortType=p1  RightPortType=p1  LConnTagsString=A|B|C  RConnTagsString=A|B|C  BranchType=C  Resistance=1  Inductance=1e-3  Capacitance=1/(C*2*pi*60)  Measurements=None
  Three-Phase Series RLC Branch3 : powerlib/Elements/Three-Phase Series RLC Branch  DialogController=POWERSYS.PowerSysDialog  PhysicalDomain=powersysdomain  SubClassName=unknown  LeftPortType=p1  RightPortType=p1  LConnTagsString=A|B|C  RConnTagsString=A|B|C  BranchType=RL  Resistance=R  Inductance=L/(2*pi*60)  Capacitance=1/(336*2*pi*60)  Measurements=None
  A* : PMIOPort  Tag=PMCPort  Port=1  Side=Right
  B* : PMIOPort  Tag=PMCPort  Port=2  Side=Right
  C* : PMIOPort  Tag=PMCPort  Port=3  Side=Right
  A : PMIOPort  Tag=PMCPort  Port=4  Side=Left
  B : PMIOPort  Tag=PMCPort  Port=5  Side=Left
  C : PMIOPort  Tag=PMCPort  Port=6  Side=Left
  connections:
  Three-Phase Parallel RLC Branch/LConn1 -- A*/RConn1 -- Three-Phase Series RLC Branch3/LConn1
  Three-Phase Parallel RLC Branch/LConn2 -- B*/RConn1 -- Three-Phase Series RLC Branch3/LConn2
  Three-Phase Parallel RLC Branch/LConn3 -- C*/RConn1 -- Three-Phase Series RLC Branch3/LConn3
  Three-Phase Series RLC Branch3/RConn1 -- A/RConn1
  Three-Phase Series RLC Branch3/RConn2 -- B/RConn1
  Three-Phase Series RLC Branch3/RConn3 -- C/RConn1
  Ground/LConn1 -- Three-Phase Parallel RLC Branch/RConn2 -- Three-Phase Parallel RLC Branch/RConn3 -- Three-Phase Parallel RLC Branch/RConn1

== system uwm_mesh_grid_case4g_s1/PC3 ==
  3-phase  Instantaneous  Active & Reactive Power : powerlib_extras/Measurements/3-phase  Instantaneous  Active & Reactive Power  DialogController=POWERSYS.PowerSysDialog  SystemSampleTime=-1
  Ground : powerlib/Elements/Ground  DialogController=POWERSYS.PowerSysDialog  PhysicalDomain=powersysdomain  SubClassName=unknown  LeftPortType=p1  RightPortType=p1  LConnTagsString=a
  Three-Phase Parallel RLC Branch : powerlib/Elements/Three-Phase Parallel RLC Branch  DialogController=POWERSYS.PowerSysDialog  PhysicalDomain=powersysdomain  SubClassName=unknown  LeftPortType=p1  RightPortType=p1  LConnTagsString=A|B|C  RConnTagsString=A|B|C  BranchType=C  Resistance=1  Inductance=1e-3  Capacitance=1/(C*2*pi*60)  Measurements=None
  Three-Phase Series RLC Branch3 : powerlib/Elements/Three-Phase Series RLC Branch  DialogController=POWERSYS.PowerSysDialog  PhysicalDomain=powersysdomain  SubClassName=unknown  LeftPortType=p1  RightPortType=p1  LConnTagsString=A|B|C  RConnTagsString=A|B|C  BranchType=RL  Resistance=R  Inductance=L/(2*pi*60)  Capacitance=1/(336*2*pi*60)  Measurements=None
  Three-Phase V-I Measurement : powerlib/Measurements/Three-Phase V-I Measurement  DialogController=POWERSYS.PowerSysDialog  SystemSampleTime=-1  VoltageMeasurement=phase-to-ground  SetLabelV=off  LabelV=Vabc  Vpu=off  VpuLL=off  CurrentMeasurement=yes  SetLabelI=off  LabelI=Iabc  Ipu=off  Pbase=100e6  Vbase=500e3  OutputType=Complex  PhasorSimulation=off  PSBequivalent=0
  A* : PMIOPort  Tag=PMCPort  Port=1  Side=Right
  B* : PMIOPort  Tag=PMCPort  Port=2  Side=Right
  C* : PMIOPort  Tag=PMCPort  Port=3  Side=Right
  A : PMIOPort  Tag=PMCPort  Port=4  Side=Left
  B : PMIOPort  Tag=PMCPort  Port=5  Side=Left
  C : PMIOPort  Tag=PMCPort  Port=6  Side=Left
  PQ : Outport  OutDataType=fixdt(1, 16)  OutScaling=2^0
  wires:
  Three-Phase V-I Measurement/1 -> 3-phase  Instantaneous  Active & Reactive Power/1
  Three-Phase V-I Measurement/2 -> 3-phase  Instantaneous  Active & Reactive Power/2
  3-phase  Instantaneous  Active & Reactive Power/1 -> PQ/1
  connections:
  Three-Phase Parallel RLC Branch/LConn1 -- A*/RConn1 -- Three-Phase Series RLC Branch3/LConn1
  Three-Phase Parallel RLC Branch/LConn2 -- B*/RConn1 -- Three-Phase Series RLC Branch3/LConn2
  Three-Phase Parallel RLC Branch/LConn3 -- C*/RConn1 -- Three-Phase Series RLC Branch3/LConn3
  Ground/LConn1 -- Three-Phase Parallel RLC Branch/RConn2 -- Three-Phase Parallel RLC Branch/RConn1 -- Three-Phase Parallel RLC Branch/RConn3
  Three-Phase V-I Measurement/RConn2 -- Three-Phase Series RLC Branch3/RConn2
  Three-Phase V-I Measurement/RConn3 -- Three-Phase Series RLC Branch3/RConn3
  Three-Phase V-I Measurement/RConn1 -- Three-Phase Series RLC Branch3/RConn1
  A/RConn1 -- Three-Phase V-I Measurement/LConn1
  B/RConn1 -- Three-Phase V-I Measurement/LConn2
  C/RConn1 -- Three-Phase V-I Measurement/LConn3

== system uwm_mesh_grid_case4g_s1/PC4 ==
  3-phase  Instantaneous  Active & Reactive Power : powerlib_extras/Measurements/3-phase  Instantaneous  Active & Reactive Power  DialogController=POWERSYS.PowerSysDialog  SystemSampleTime=-1
  Ground : powerlib/Elements/Ground  DialogController=POWERSYS.PowerSysDialog  PhysicalDomain=powersysdomain  SubClassName=unknown  LeftPortType=p1  RightPortType=p1  LConnTagsString=a
  Three-Phase Parallel RLC Branch : powerlib/Elements/Three-Phase Parallel RLC Branch  DialogController=POWERSYS.PowerSysDialog  PhysicalDomain=powersysdomain  SubClassName=unknown  LeftPortType=p1  RightPortType=p1  LConnTagsString=A|B|C  RConnTagsString=A|B|C  BranchType=C  Resistance=1  Inductance=1e-3  Capacitance=1/(C*2*pi*60)  Measurements=None
  Three-Phase Series RLC Branch3 : powerlib/Elements/Three-Phase Series RLC Branch  DialogController=POWERSYS.PowerSysDialog  PhysicalDomain=powersysdomain  SubClassName=unknown  LeftPortType=p1  RightPortType=p1  LConnTagsString=A|B|C  RConnTagsString=A|B|C  BranchType=RL  Resistance=R  Inductance=L/(2*pi*60)  Capacitance=1/(336*2*pi*60)  Measurements=None
  Three-Phase V-I Measurement : powerlib/Measurements/Three-Phase V-I Measurement  DialogController=POWERSYS.PowerSysDialog  SystemSampleTime=-1  VoltageMeasurement=phase-to-ground  SetLabelV=off  LabelV=Vabc  Vpu=off  VpuLL=off  CurrentMeasurement=yes  SetLabelI=off  LabelI=Iabc  Ipu=off  Pbase=100e6  Vbase=500e3  OutputType=Complex  PhasorSimulation=off  PSBequivalent=0
  A* : PMIOPort  Tag=PMCPort  Port=1  Side=Right
  B* : PMIOPort  Tag=PMCPort  Port=2  Side=Right
  C* : PMIOPort  Tag=PMCPort  Port=3  Side=Right
  A : PMIOPort  Tag=PMCPort  Port=4  Side=Left
  B : PMIOPort  Tag=PMCPort  Port=5  Side=Left
  C : PMIOPort  Tag=PMCPort  Port=6  Side=Left
  PQ : Outport  OutDataType=fixdt(1, 16)  OutScaling=2^0
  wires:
  Three-Phase V-I Measurement/1 -> 3-phase  Instantaneous  Active & Reactive Power/1
  Three-Phase V-I Measurement/2 -> 3-phase  Instantaneous  Active & Reactive Power/2
  3-phase  Instantaneous  Active & Reactive Power/1 -> PQ/1
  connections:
  A*/RConn1 -- Three-Phase Series RLC Branch3/LConn1 -- Three-Phase Parallel RLC Branch/LConn1
  B*/RConn1 -- Three-Phase Series RLC Branch3/LConn2 -- Three-Phase Parallel RLC Branch/LConn2
  C*/RConn1 -- Three-Phase Series RLC Branch3/LConn3 -- Three-Phase Parallel RLC Branch/LConn3
  Ground/LConn1 -- Three-Phase Parallel RLC Branch/RConn2 -- Three-Phase Parallel RLC Branch/RConn3 -- Three-Phase Parallel RLC Branch/RConn1
  Three-Phase V-I Measurement/RConn1 -- Three-Phase Series RLC Branch3/RConn1
  Three-Phase V-I Measurement/RConn2 -- Three-Phase Series RLC Branch3/RConn2
  Three-Phase V-I Measurement/RConn3 -- Three-Phase Series RLC Branch3/RConn3
  A/RConn1 -- Three-Phase V-I Measurement/LConn1
  B/RConn1 -- Three-Phase V-I Measurement/LConn2
  C/RConn1 -- Three-Phase V-I Measurement/LConn3

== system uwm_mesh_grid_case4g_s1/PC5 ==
  3-phase  Instantaneous  Active & Reactive Power : powerlib_extras/Measurements/3-phase  Instantaneous  Active & Reactive Power  DialogController=POWERSYS.PowerSysDialog  SystemSampleTime=-1
  Ground : powerlib/Elements/Ground  DialogController=POWERSYS.PowerSysDialog  PhysicalDomain=powersysdomain  SubClassName=unknown  LeftPortType=p1  RightPortType=p1  LConnTagsString=a
  Three-Phase Parallel RLC Branch : powerlib/Elements/Three-Phase Parallel RLC Branch  DialogController=POWERSYS.PowerSysDialog  PhysicalDomain=powersysdomain  SubClassName=unknown  LeftPortType=p1  RightPortType=p1  LConnTagsString=A|B|C  RConnTagsString=A|B|C  BranchType=C  Resistance=1  Inductance=1e-3  Capacitance=1/(C*2*pi*60)  Measurements=None
  Three-Phase Series RLC Branch3 : powerlib/Elements/Three-Phase Series RLC Branch  DialogController=POWERSYS.PowerSysDialog  PhysicalDomain=powersysdomain  SubClassName=unknown  LeftPortType=p1  RightPortType=p1  LConnTagsString=A|B|C  RConnTagsString=A|B|C  BranchType=RL  Resistance=R  Inductance=L/(2*pi*60)  Capacitance=1/(336*2*pi*60)  Measurements=None
  Three-Phase V-I Measurement : powerlib/Measurements/Three-Phase V-I Measurement  DialogController=POWERSYS.PowerSysDialog  SystemSampleTime=-1  VoltageMeasurement=phase-to-ground  SetLabelV=off  LabelV=Vabc  Vpu=off  VpuLL=off  CurrentMeasurement=yes  SetLabelI=off  LabelI=Iabc  Ipu=off  Pbase=100e6  Vbase=500e3  OutputType=Complex  PhasorSimulation=off  PSBequivalent=0
  A* : PMIOPort  Tag=PMCPort  Port=1  Side=Right
  B* : PMIOPort  Tag=PMCPort  Port=2  Side=Right
  C* : PMIOPort  Tag=PMCPort  Port=3  Side=Right
  A : PMIOPort  Tag=PMCPort  Port=4  Side=Left
  B : PMIOPort  Tag=PMCPort  Port=5  Side=Left
  C : PMIOPort  Tag=PMCPort  Port=6  Side=Left
  PQ : Outport  OutDataType=fixdt(1, 16)  OutScaling=2^0
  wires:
  Three-Phase V-I Measurement/1 -> 3-phase  Instantaneous  Active & Reactive Power/1
  Three-Phase V-I Measurement/2 -> 3-phase  Instantaneous  Active & Reactive Power/2
  3-phase  Instantaneous  Active & Reactive Power/1 -> PQ/1
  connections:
  Three-Phase Parallel RLC Branch/LConn1 -- A*/RConn1 -- Three-Phase Series RLC Branch3/LConn1
  Three-Phase Parallel RLC Branch/LConn2 -- B*/RConn1 -- Three-Phase Series RLC Branch3/LConn2
  Three-Phase Parallel RLC Branch/LConn3 -- C*/RConn1 -- Three-Phase Series RLC Branch3/LConn3
  Ground/LConn1 -- Three-Phase Parallel RLC Branch/RConn2 -- Three-Phase Parallel RLC Branch/RConn3 -- Three-Phase Parallel RLC Branch/RConn1
  Three-Phase V-I Measurement/RConn1 -- Three-Phase Series RLC Branch3/RConn1
  Three-Phase V-I Measurement/RConn2 -- Three-Phase Series RLC Branch3/RConn2
  Three-Phase V-I Measurement/RConn3 -- Three-Phase Series RLC Branch3/RConn3
  A/RConn1 -- Three-Phase V-I Measurement/LConn1
  B/RConn1 -- Three-Phase V-I Measurement/LConn2
  C/RConn1 -- Three-Phase V-I Measurement/LConn3

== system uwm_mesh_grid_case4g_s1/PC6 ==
  3-phase  Instantaneous  Active & Reactive Power : powerlib_extras/Measurements/3-phase  Instantaneous  Active & Reactive Power  DialogController=POWERSYS.PowerSysDialog  SystemSampleTime=-1
  Ground : powerlib/Elements/Ground  DialogController=POWERSYS.PowerSysDialog  PhysicalDomain=powersysdomain  SubClassName=unknown  LeftPortType=p1  RightPortType=p1  LConnTagsString=a
  Three-Phase Parallel RLC Branch : powerlib/Elements/Three-Phase Parallel RLC Branch  DialogController=POWERSYS.PowerSysDialog  PhysicalDomain=powersysdomain  SubClassName=unknown  LeftPortType=p1  RightPortType=p1  LConnTagsString=A|B|C  RConnTagsString=A|B|C  BranchType=C  Resistance=1  Inductance=1e-3  Capacitance=1/(C*2*pi*60)  Measurements=None
  Three-Phase Series RLC Branch3 : powerlib/Elements/Three-Phase Series RLC Branch  DialogController=POWERSYS.PowerSysDialog  PhysicalDomain=powersysdomain  SubClassName=unknown  LeftPortType=p1  RightPortType=p1  LConnTagsString=A|B|C  RConnTagsString=A|B|C  BranchType=RL  Resistance=R  Inductance=L/(2*pi*60)  Capacitance=1/(336*2*pi*60)  Measurements=None
  Three-Phase V-I Measurement : powerlib/Measurements/Three-Phase V-I Measurement  DialogController=POWERSYS.PowerSysDialog  SystemSampleTime=-1  VoltageMeasurement=phase-to-ground  SetLabelV=off  LabelV=Vabc  Vpu=off  VpuLL=off  CurrentMeasurement=yes  SetLabelI=off  LabelI=Iabc  Ipu=off  Pbase=100e6  Vbase=500e3  OutputType=Complex  PhasorSimulation=off  PSBequivalent=0
  A* : PMIOPort  Tag=PMCPort  Port=1  Side=Right
  B* : PMIOPort  Tag=PMCPort  Port=2  Side=Right
  C* : PMIOPort  Tag=PMCPort  Port=3  Side=Right
  A : PMIOPort  Tag=PMCPort  Port=4  Side=Left
  B : PMIOPort  Tag=PMCPort  Port=5  Side=Left
  C : PMIOPort  Tag=PMCPort  Port=6  Side=Left
  PQ : Outport  OutDataType=fixdt(1, 16)  OutScaling=2^0
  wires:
  Three-Phase V-I Measurement/1 -> 3-phase  Instantaneous  Active & Reactive Power/1
  Three-Phase V-I Measurement/2 -> 3-phase  Instantaneous  Active & Reactive Power/2
  3-phase  Instantaneous  Active & Reactive Power/1 -> PQ/1
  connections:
  Three-Phase Parallel RLC Branch/LConn1 -- A*/RConn1 -- Three-Phase Series RLC Branch3/LConn1
  Three-Phase Parallel RLC Branch/LConn2 -- B*/RConn1 -- Three-Phase Series RLC Branch3/LConn2
  Three-Phase Parallel RLC Branch/LConn3 -- C*/RConn1 -- Three-Phase Series RLC Branch3/LConn3
  Ground/LConn1 -- Three-Phase Parallel RLC Branch/RConn2 -- Three-Phase Parallel RLC Branch/RConn3 -- Three-Phase Parallel RLC Branch/RConn1
  Three-Phase V-I Measurement/RConn1 -- Three-Phase Series RLC Branch3/RConn1
  Three-Phase V-I Measurement/RConn2 -- Three-Phase Series RLC Branch3/RConn2
  Three-Phase V-I Measurement/RConn3 -- Three-Phase Series RLC Branch3/RConn3
  A/RConn1 -- Three-Phase V-I Measurement/LConn1
  B/RConn1 -- Three-Phase V-I Measurement/LConn2
  C/RConn1 -- Three-Phase V-I Measurement/LConn3

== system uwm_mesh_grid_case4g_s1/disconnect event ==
  Step1 : Step  Time=[tstart]  Before=1  After=0  SampleTime=0
  Step2 : Step  Time=[tstop]  SampleTime=0
  Sum : Sum  OutDataType=fixdt(1, 16)  OutScaling=2^0
  Out1 : Outport
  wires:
  Step2/1 -> Sum/2
  Step1/1 -> Sum/1
  Sum/1 -> Out1/1

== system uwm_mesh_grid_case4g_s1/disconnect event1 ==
  Step1 : Step  Time=[tstart]  Before=1  After=0  SampleTime=0
  Step2 : Step  Time=[tstop]  SampleTime=0
  Sum : Sum  OutDataType=fixdt(1, 16)  OutScaling=2^0
  Out1 : Outport
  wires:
  Step2/1 -> Sum/2
  Step1/1 -> Sum/1
  Sum/1 -> Out1/1

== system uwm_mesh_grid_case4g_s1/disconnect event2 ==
  Step1 : Step  Time=[tstart]  Before=1  After=0  SampleTime=0
  Step2 : Step  Time=[tstop]  SampleTime=0
  Sum : Sum  OutDataType=fixdt(1, 16)  OutScaling=2^0
  Out1 : Outport
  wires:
  Step2/1 -> Sum/2
  Step1/1 -> Sum/1
  Sum/1 -> Out1/1
